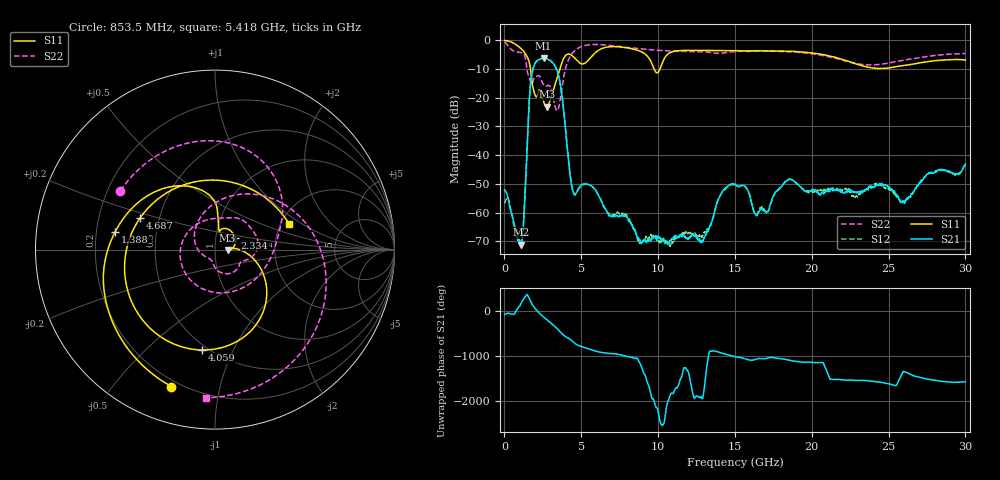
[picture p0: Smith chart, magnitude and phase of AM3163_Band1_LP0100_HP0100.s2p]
!Agilent Technologies,E8364B,MY43040894,A.07.50.67
!Agilent E8364B: A.07.50.67
!Date: Thursday, August 20, 2020 11:18:07
!Correction: S11(Full 2 Port(1,2))
!S21(Full 2 Port(1,2))
!S12(Full 2 Port(1,2))
!S22(Full 2 Port(1,2))
!S2P File: Measurements: S11, S21, S12, S22:
# Hz S  dB  R 50
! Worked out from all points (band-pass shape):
!   3201 points, 10 MHz to 30 GHz, reference 50 ohm
!   highest |S21| = -6.29 dB at 2.55 GHz (marker M1); lowest = -71.1 dB at 1.078 GHz (marker M2)
!   |S21| within 3 dB of the highest: 1.898 GHz to 3.323 GHz (1.425 GHz wide, 54.6 % of centre)
!   lowest |S11| = -23.1 dB at 2.747 GHz (marker M3), VSWR 1.15, Z = 57.5 - j0.288 ohm
!   |S11| at or under -10 dB: 1.694 GHz to 3.608 GHz (1.914 GHz wide, 72.2 % of centre); 9.736 GHz to 10.12 GHz (387.9 MHz wide, 3.91 % of centre)
!   |S22| runs from -24.6 to -0.6 dB; largest |S21 - S12| = 0.005
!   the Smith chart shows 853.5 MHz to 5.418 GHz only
!   S11 on the Smith chart (normalised r, x): 853.5 MHz: 0.17, -0.72; 1.388 GHz: 0.28, +0.08; 2.334 GHz: 1.24, +0.17; 4.059 GHz: 0.47, -0.77; 4.687 GHz: 0.39, +0.17; 5.418 GHz: 2.23, +0.78
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1e7  -0.10 -8.1  -52.08 -81.1  -56.81 -60.1  -0.59 -26.0
8.534688e8  -1.93 -107.6  -68.11 51.8  -69.38 -13.4  -4.15 148.2
1.078394e9  -2.91 -138.7  -71.07 166.2  -70.06 -10.9  -4.24 109.0
1.387666e9  -4.94 170.2  -48.96 -32.4  -48.12 -42.3  -7.06 31.8
1.753169e9  -12.96 86.8  -12.75 173.6  -12.76 173.5  -15.14 131.3
2.334225e9  -17.74 30.9  -6.54 -72.9  -6.54 -73.0  -13.01 -5.5
2.549778e9  -21.47 -2.2  -6.29 -137.4  -6.29 -137.5  -15.50 -22.0
2.746588e9  -23.11 -2.0  -6.47 166.9  -6.48 166.8  -15.96 -30.2
3.449478e9  -12.75 -15.0  -10.95 -42.5  -10.96 -42.4  -24.48 -127.3
4.05865e9  -4.98 -97.3  -35.76 132.9  -35.64 133.1  -8.31 53.0
4.686566e9  -6.88 157.1  -53.00 -24.5  -53.27 -26.3  -3.14 -32.0
5.014581e9  -8.21 95.1  -50.28 -72.7  -50.58 -74.7  -2.20 -62.3
5.417572e9  -7.18 18.9  -50.19 -117.2  -50.13 -118.0  -1.66 -93.3
6.345388e9  -2.90 -93.3  -56.36 157.7  -56.15 156.1  -1.57 -149.4
7.451269e9  -2.30 -170.2  -61.32 116.9  -60.23 117.2  -2.17 158.8
1.000979e10  -11.13 100.0  -68.14 -72.7  -69.78 31.5  -3.54 59.7
1.242773e10  -3.54 6.6  -67.79 -96.9  -67.19 180.0  -3.96 -22.8
1.5005e10  -3.65 -72.0  -50.16 67.0  -50.39 68.5  -3.95 -90.2
2.000958e10  -4.44 163.5  -52.07 -58.3  -52.58 -59.1  -4.70 136.9
2.275554e10  -8.03 60.5  -52.86 -95.3  -53.96 -106.2  -7.98 21.4
2.500479e10  -9.66 -62.1  -51.08 -174.0  -51.66 -171.1  -7.96 -92.1
3e10  -6.92 104.8  -43.08 -128.0  -42.94 -130.6  -4.63 102.8
